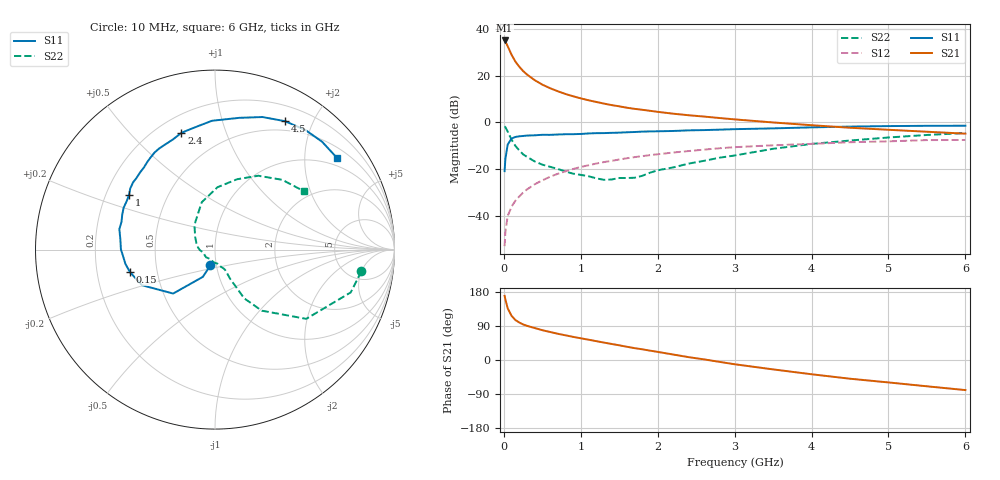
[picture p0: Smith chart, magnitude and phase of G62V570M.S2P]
! SIEMENS Small Signal Semiconductors
! BFG193
! Si NPN RF Bipolar Junction Transistor in SOT223
! VCE = 2.5 V  IC = 70 mA
! Common Emitter S-Parameters:  August  1996
# GHz  S  MA  R  50
!  f  S11  S21  S12  S22
! GHz  MAG  ANG  MAG  ANG  MAG  ANG  MAG  ANG
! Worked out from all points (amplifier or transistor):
!   36 points, 10 MHz to 6 GHz, reference 50 ohm
!   highest |S21| = 35.0 dB at 10 MHz (marker M1)
!   |S21| within 3 dB of that: start of sweep to 57.59 MHz
!   unconditionally stable (mu >= 1): start of sweep to 13.07 MHz; 248.7 MHz to 2.606 GHz
!   at 250 MHz: K = 1.00, MAG = 25.7 dB, |S12| = -29.9 dB
!   at 1.4 GHz: K = 1.08, MAG = 10.2 dB, |S12| = -16.4 dB
!   at 6 GHz: K = 0.95, MSG = 1.3 dB, |S12| = -7.5 dB
!   S11 on the Smith chart (normalised r, x): 10 MHz: 0.94, -0.17; 150 MHz: 0.35, -0.11; 1 GHz: 0.30, +0.27; 2.4 GHz: 0.30, +0.71; 4.5 GHz: 0.38, +1.62; 6 GHz: 0.76, +2.80
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0.01  0.0915 -106.1  55.91 169.3  0.0023 80.7  0.8244 -8.5
0.02  0.1666 -114.1  53.24 159.8  0.0046 74.1  0.793 -17.5
0.05  0.3382 -133.6  42.17 136.5  0.0101 69.1  0.6381 -37.2
0.1  0.4525 -154.0  27.8 116.7  0.016 65.6  0.4283 -52.6
0.15  0.4903 -165.2  19.86 105.4  0.0214 66.2  0.3158 -59.1
0.2  0.5055 -171.0  15.44 99.0  0.0263 68.8  0.2543 -60.2
0.25  0.5143 -176.3  12.5 93.9  0.0319 69.5  0.2088 -61.6
0.3  0.5243 179.8  10.54 90.2  0.0372 69.7  0.185 -62.6
0.4  0.5311 173.4  7.983 84.4  0.0479 70.0  0.1476 -63.0
0.5  0.5451 167.9  6.4 78.7  0.0581 69.0  0.1259 -63.5
0.6  0.5433 163.5  5.373 74.0  0.0693 68.2  0.1133 -66.1
0.8  0.5599 155.3  4.043 65.2  0.0905 64.3  0.0899 -74.6
1  0.5679 147.4  3.259 57.3  0.1123 60.8  0.0761 -85.8
1.1  0.5823 144.2  2.969 53.6  0.122 59.0  0.0713 -95.8
1.3  0.5922 137.6  2.522 46.0  0.1426 54.7  0.0597 -115.7
1.6  0.6167 127.8  2.058 34.9  0.1724 47.6  0.0653 -150.1
2.2  0.657 110.9  1.536 14.5  0.2281 33.5  0.1096 160.9
2.4  0.6772 106.0  1.424 7.6  0.2452 29.2  0.1324 146.9
3.5  0.7467 79.5  0.998 -24.8  0.3254 1.4  0.2742 105.6
4.5  0.8149 61.4  0.77 -49.4  0.3781 -18.8  0.4112 72.5
5.5  0.8469 45.2  0.633 -69.4  0.42 -42.3  0.5403 46.0
6  0.85 37.1  0.576 -79.4  0.4224 -55.7  0.5936 33.1
